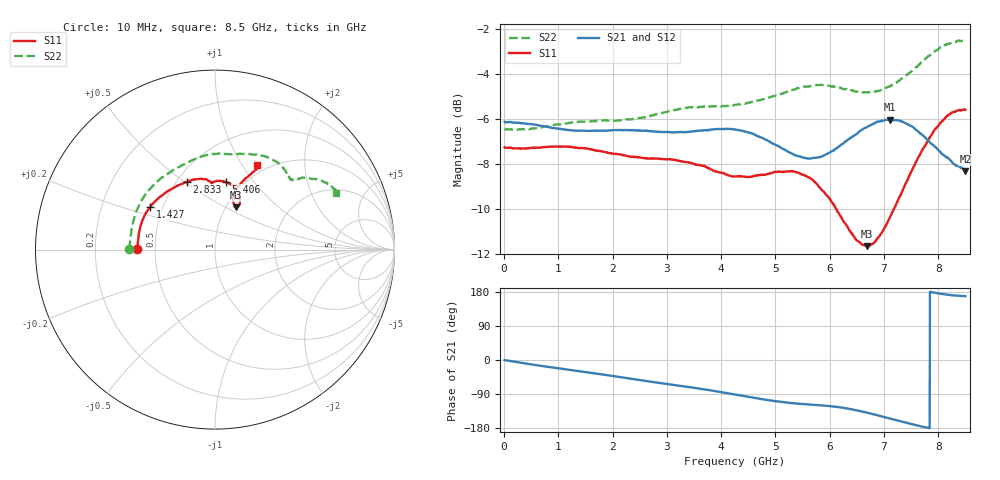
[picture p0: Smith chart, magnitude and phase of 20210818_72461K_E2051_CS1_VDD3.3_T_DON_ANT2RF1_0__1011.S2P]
!Agilent Technologies,E5071C,MY46417908,A.11.23
!Date: Wed Aug 18 14:24:35 2021
!Data & Calibration Information:
!Freq	S11:SOLT2(ON)	S21:SOLT2(ON)	S12:SOLT2(ON)	S22:SOLT2(ON)
!PortZ  Port1:50+j0  Port2:50+j0
!Above PortZ is port z conversion or system Z0 setting when saving the data.
!When reading, reference impedance value at option line is always used.
# Hz S dB R 50
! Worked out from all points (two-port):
!   1601 points, 10 MHz to 8.5 GHz, reference 50 ohm
!   highest |S21| = -6.02 dB at 7.115 GHz (marker M1); lowest = -8.3 dB at 8.5 GHz (marker M2)
!   |S21| within 3 dB of the highest: start of sweep to end of sweep
!   lowest |S11| = -11.6 dB at 6.691 GHz (marker M3), VSWR 1.71, Z = 55.6 + j28.1 ohm
!   |S11| at or under -10 dB: 6.124 GHz to 7.178 GHz (1.054 GHz wide, 15.9 % of centre)
!   |S22| runs from -6.5 to -2.5 dB; largest |S21 - S12| = 0.0025
!   S11 on the Smith chart (normalised r, x): 10 MHz: 0.39, +0.00; 1.427 GHz: 0.43, +0.25; 2.833 GHz: 0.56, +0.51; 5.406 GHz: 0.83, +0.73; 8.5 GHz: 0.90, +1.17
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1e7  -7.25 179.7  -6.11 -0.4  -6.11 -0.3  -6.42 179.6
7.900188e8  -7.24 162.4  -6.34 -17.9  -6.34 -17.9  -6.32 158.5
1.426769e9  -7.28 146.5  -6.50 -30.5  -6.51 -30.5  -6.10 140.0
2.1325e9  -7.56 128.7  -6.48 -44.9  -6.48 -44.9  -6.05 120.0
2.832925e9  -7.75 112.5  -6.56 -59.9  -6.56 -60.0  -5.76 103.6
2.843538e9  -7.75 112.3  -6.55 -60.1  -6.55 -60.2  -5.75 103.4
3.61825e9  -8.04 97.8  -6.50 -76.1  -6.49 -76.1  -5.45 88.8
4.255e9  -8.54 93.0  -6.46 -91.2  -6.45 -91.2  -5.36 80.2
4.8493e9  -8.44 90.3  -6.94 -105.5  -6.94 -105.5  -5.05 72.6
5.406456e9  -8.37 81.0  -7.63 -115.0  -7.64 -115.0  -4.62 62.7
5.671769e9  -8.67 74.4  -7.73 -117.9  -7.75 -117.9  -4.52 57.4
6.085656e9  -9.84 64.6  -7.36 -123.1  -7.37 -123.2  -4.54 49.7
6.404031e9  -11.07 61.3  -6.80 -130.2  -6.79 -130.3  -4.71 45.2
6.690569e9  -11.64 63.7  -6.34 -139.2  -6.33 -139.2  -4.81 42.7
6.849756e9  -11.41 66.6  -6.15 -144.8  -6.16 -144.8  -4.77 42.3
7.088538e9  -10.47 70.2  -6.02 -153.7  -6.03 -153.7  -4.55 41.3
7.115069e9  -10.33 70.4  -6.02 -154.7  -6.03 -154.6  -4.52 41.3
7.3114e9  -9.34 71.1  -6.09 -162.1  -6.09 -162.1  -4.22 40.0
7.502425e9  -8.33 69.4  -6.30 -168.9  -6.31 -169.0  -3.88 38.7
7.873862e9  -6.70 64.8  -7.09 179.2  -7.06 179.1  -3.11 33.5
8.165706e9  -5.84 62.7  -7.70 172.4  -7.68 172.4  -2.66 29.2
8.5e9  -5.58 63.4  -8.30 168.4  -8.26 168.5  -2.55 25.2
